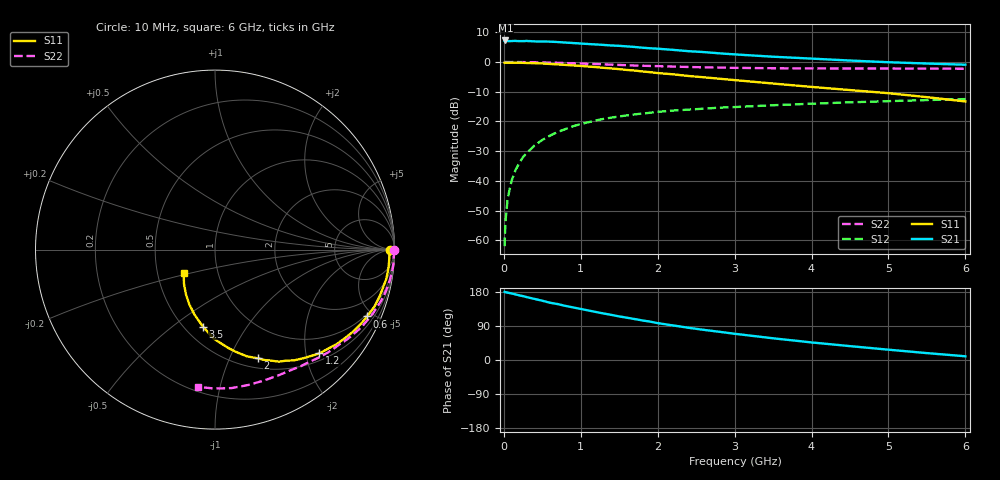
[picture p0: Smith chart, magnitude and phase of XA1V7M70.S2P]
! SIEMENS Discrete & RF Semiconductors
! BFY180
! Si NPN RF Bipolar Junction Transistor in MICRO-X
! VCE = 1.75 V  IC = 0.7 mA
! Common Emitter S-Parameters:  May  1997
# GHz  S  MA  R  50
!  f  S11  S21  S12  S22
! GHz  MAG  ANG  MAG  ANG  MAG  ANG  MAG  ANG
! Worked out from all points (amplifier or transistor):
!   36 points, 10 MHz to 6 GHz, reference 50 ohm
!   highest |S21| = 7.2 dB at 20 MHz (marker M1)
!   |S21| within 3 dB of that: start of sweep to 2.117 GHz
!   unconditionally stable (mu >= 1): 4.22 GHz to end of sweep
!   at 250 MHz: K = 0.08, MSG = 19.5 dB, |S12| = -31.9 dB
!   at 1.4 GHz: K = 0.46, MSG = 12.1 dB, |S12| = -18.7 dB
!   at 6 GHz: K = 1.06, MAG = 4.3 dB, |S12| = -12.5 dB
!   S11 on the Smith chart (normalised r, x): 10 MHz: 72, -9; 600 MHz: 0.88, -4.61; 1.2 GHz: 0.64, -2.27; 2 GHz: 0.61, -1.28; 3.5 GHz: 0.61, -0.65; 6 GHz: 0.68, -0.19
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0.01  0.9729 -0.2  2.248 179.8  0.0008 87.3  0.997 -0.2
0.02  0.9696 -0.8  2.302 178.9  0.002 93.5  0.9999 -0.5
0.05  0.9722 -1.9  2.249 177.8  0.0051 82.7  0.9972 -1.3
0.1  0.9722 -4.0  2.251 175.6  0.01 89.2  0.9962 -2.5
0.15  0.9718 -6.1  2.261 173.2  0.0151 87.0  0.998 -3.7
0.25  0.9677 -10.0  2.242 168.5  0.0253 82.7  0.9956 -6.3
0.3  0.9618 -11.9  2.259 165.8  0.0296 81.1  0.9924 -7.5
0.4  0.9539 -15.7  2.22 161.1  0.0396 78.9  0.989 -9.9
0.6  0.9264 -23.7  2.2 151.1  0.0578 73.0  0.9763 -14.7
0.8  0.8934 -31.0  2.12 142.7  0.0744 67.1  0.9582 -19.4
1.1  0.8378 -41.2  2.005 130.7  0.0971 59.6  0.9315 -25.8
1.2  0.8204 -44.8  1.971 126.6  0.1044 57.3  0.923 -28.0
1.5  0.7581 -54.5  1.869 115.0  0.1214 50.8  0.8922 -33.7
2  0.6516 -68.4  1.674 97.3  0.1452 42.3  0.8517 -42.2
2.2  0.6206 -73.4  1.599 91.2  0.1525 39.0  0.838 -45.4
2.6  0.5532 -82.3  1.468 79.5  0.1641 34.1  0.8131 -51.1
3  0.4962 -90.8  1.342 69.2  0.1747 29.6  0.7968 -56.6
3.5  0.4342 -98.9  1.227 57.3  0.1875 24.9  0.7849 -63.0
4  0.3812 -107.3  1.14 46.4  0.199 20.3  0.7788 -69.6
4.5  0.3373 -115.1  1.058 36.6  0.2097 16.0  0.7767 -76.3
5.5  0.2562 -132.5  0.942 18.2  0.229 7.8  0.7741 -90.2
6  0.217 -143.3  0.9 9.8  0.2379 3.3  0.7705 -97.1
